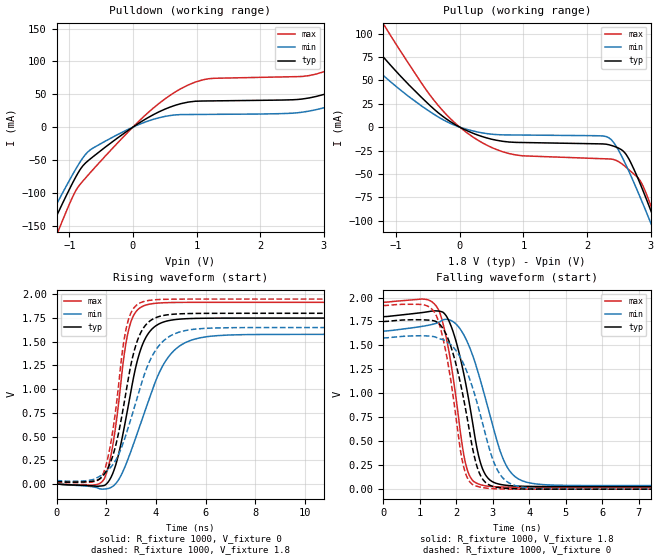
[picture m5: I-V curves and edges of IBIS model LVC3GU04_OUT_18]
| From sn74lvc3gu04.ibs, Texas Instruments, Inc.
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[Model]   LVC3GU04_OUT_18
Model_type  Output
Vref =   0
Rref =   1000
Cref =   30p
Vmeas =   0.9
| variable   typ   min   max
C_comp   10.62pF   7.07pF   15.30pF
| C_pullup   10.42pF   7.25pF   12.72pF
| C_pulldown   10.81pF   7.07pF   15.30pF
[Temperature Range]   40   100   -40
| Ambient temperature   25   85   -40
[Voltage range]   1.8   1.65   1.95
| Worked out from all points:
|   slope of the pulldown table from 0 to 0.27 V, typ, clamps not added: 16.6 ohm
|   slope of the pullup table from 0 to 0.27 V, typ, clamps not added: 33.1 ohm
|   rising waveform, R_fixture 1000, V_fixture 0: 20-80 % time 834ps typ, 1.36ns min, 580ps max; typ from 0 V to 1.75 V
|   falling waveform, R_fixture 1000, V_fixture 1.8: 20-80 % time 531ps typ, 730ps min, 451ps max; typ from 1.8 V to 0.027 V
|   rising waveform, R_fixture 1000, V_fixture 1.8: 20-80 % time 816ps typ, 1.23ns min, 583ps max; typ from 0.027 V to 1.8 V
|   falling waveform, R_fixture 1000, V_fixture 0: 20-80 % time 568ps typ, 745ps min, 463ps max; typ from 1.75 V to 0 V
[Pulldown]
| LVC3GU04_OUT_18
|   Voltage   I(typ)   I(min)   I(max)
-5.5V     -1.024A    -932.8mA   -1.173A
-1.5V     -197.8mA   -173.7mA   -237mA
-1.22V    -139.5mA   -121.3mA   -169.4mA
-870mV    -71.15mA   -59.34mA   -92.41mA
-665mV    -48.08mA   -34.31mA   -68.79mA
670mV     33.41mA    18.66mA    53.83mA
1.195V    39.91mA    19.44mA    73.76mA
2.88V     46.7mA     26.58mA    80.85mA
4.12V     103.8mA    75.37mA    153.2mA
4.815V    154.3mA    117.5mA    219.8mA
5.435V    207.1mA    161.6mA    289.8mA
11V       864.7mA    712.8mA    1.162A
[Pullup]
| LVC3GU04_OUT_18
|   Voltage   I(typ)   I(min)   I(max)
-5.5V     528.9mA    421.5mA    733.8mA
-1.985V   141.7mA    107.2mA    204.6mA
-1.575V   105.5mA    78.75mA    153.7mA
-1.2V     74.83mA    55.07mA    110.3mA
-340mV    15.48mA    10.96mA    23.3mA
350mV     -10.02mA   -6.091mA   -16.53mA
2.345V    -18.84mA   -11.41mA   -33.99mA
2.635V    -31.3mA    -43.77mA   -44.13mA
2.85V     -62.85mA   -77.27mA   -58.89mA
3.045V    -96.52mA   -109.6mA   -91.62mA
3.135V    -112.7mA   -125mA     -109mA
11V       -1.709A    -1.61A     -1.884A
[Ramp]
| LVC3GU04_OUT_18
| variable   typ   min   max
dV/dt_r   1.06/8.44E-10   0.98/1.40E-09   1.16/5.90E-10
dV/dt_f   1.10/5.59E-10   1.04/7.99E-10   1.18/4.65E-10
R_load = 1000
[Rising Waveform]
| LVC3GU04_OUT_18
R_fixture =   1000
C_fixture =   0
L_fixture =   0
V_fixture =   0
V_fixture_min = 0
V_fixture_max = 0
|   Time   V(typ)   V(min)   V(max)
0s        32.52pV    7.411nV    2.092nV
1.925ns   -14.85mV   -52.42mV   57.23mV
2.285ns   125.4mV    -20.22mV   439.3mV
2.715ns   582.2mV    156.8mV    1.345V
2.905ns   847.6mV    281.3mV    1.628V
3.26ns    1.306V     541.6mV    1.835V
3.615ns   1.554V     809.8mV    1.888V
4.595ns   1.727V     1.369V     1.913V
6.04ns    1.748V     1.553V     1.915V
24.99ns   1.749V     1.578V     1.915V
[Falling Waveform]
| LVC3GU04_OUT_18
R_fixture =   1000
C_fixture =   0
L_fixture =   0
V_fixture =   1.8
V_fixture_min = 1.65
V_fixture_max = 1.95
|   Time   V(typ)   V(min)   V(max)
0s        1.8V       1.65V      1.95V
1.3ns     1.857V     1.716V     1.963V
1.53ns    1.858V     1.744V     1.858V
1.725ns   1.808V     1.772V     1.581V
2.265ns   1.088V     1.566V     251mV
2.58ns    402.2mV    1.241V     58.81mV
2.765ns   174.4mV    993.9mV    37.46mV
3.395ns   39.4mV     230.6mV    21.35mV
4.21ns    28.04mV    53.35mV    19.83mV
24.99ns   26.95mV    37.1mV     19.71mV
[Rising Waveform]
| LVC3GU04_OUT_18
R_fixture =   1000
C_fixture =   0
L_fixture =   0
V_fixture =   1.8
V_fixture_min = 1.65
V_fixture_max = 1.95
|   Time   V(typ)   V(min)   V(max)
0s        26.95mV    37.1mV     19.71mV
1.86ns    83.16mV    100.3mV    98.02mV
2.23ns    269.9mV    191.9mV    502.1mV
2.655ns   753.5mV    412.3mV    1.403V
2.83ns    1.018V     547.4mV    1.668V
3.145ns   1.42V      817.4mV    1.866V
3.505ns   1.647V     1.13V      1.923V
4.315ns   1.778V     1.511V     1.947V
5.645ns   1.799V     1.635V     1.95V
24.99ns   1.8V       1.65V      1.95V
[Falling Waveform]
| LVC3GU04_OUT_18
R_fixture =   1000
C_fixture =   0
L_fixture =   0
V_fixture =   0
V_fixture_min = 0
V_fixture_max = 0
|   Time   V(typ)   V(min)   V(max)
0s        1.749V     1.578V     1.915V
1.075ns   1.767V     1.601V     1.926V
1.43ns    1.752V     1.587V     1.829V
1.745ns   1.596V     1.538V     1.37V
2.215ns   914.1mV    1.294V     213.3mV
2.495ns   341.6mV    999.3mV    39.04mV
2.69ns    123.7mV    731.7mV    18.62mV
3.205ns   14.53mV    151.5mV    2.43mV
4.01ns    1.251mV    12.13mV    168.1uV
24.99ns   5.14nV     18.85nV    3.827nV
